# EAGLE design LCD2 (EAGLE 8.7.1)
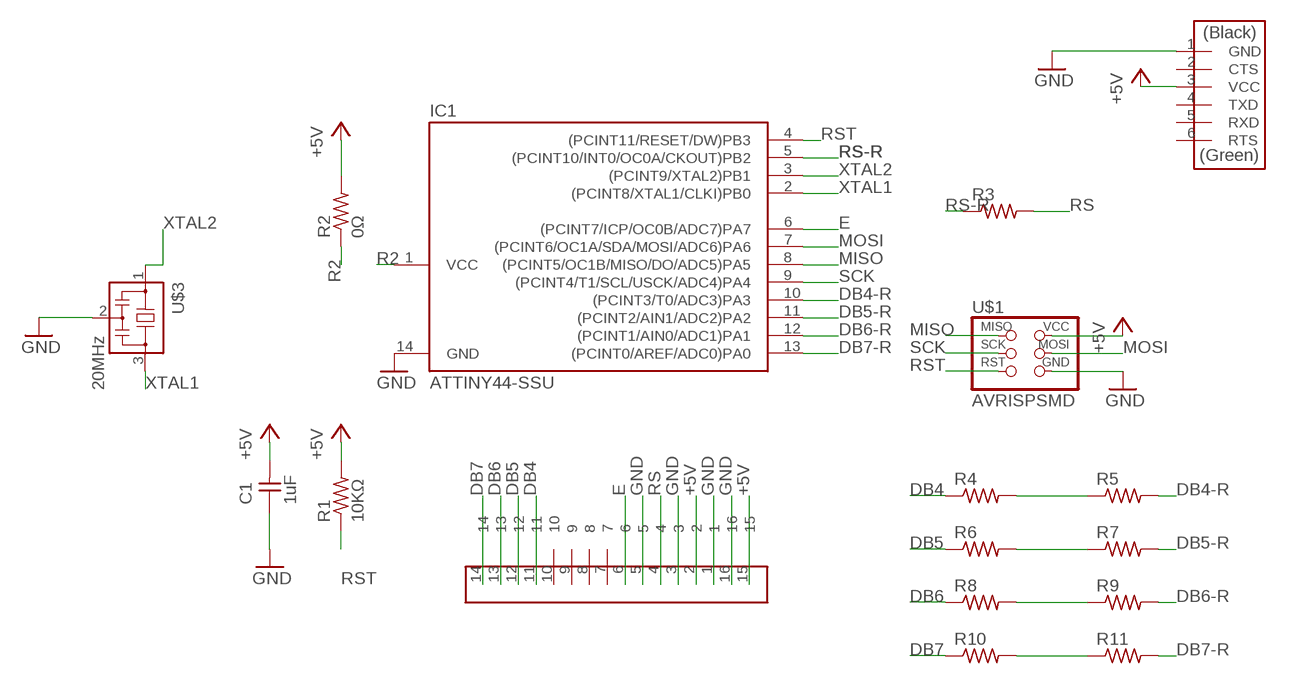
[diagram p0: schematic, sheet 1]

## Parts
C1  1uF  CAP-UNPOLARIZEDFAB  [C1206FAB]
IC1  ATTINY44-SSU  [SOIC14]
LCD1  LCD16PIN  [16PIN]
R1  10KΩ  RES-US1206FAB  [R1206FAB]
R2  0Ω  RES-US1206FAB  [R1206FAB]
R3  RES-US1206FAB  [R1206FAB]
R4  RES-US1206FAB  [R1206FAB]
R5  RES-US1206FAB  [R1206FAB]
R6  RES-US1206FAB  [R1206FAB]
R7  RES-US1206FAB  [R1206FAB]
R8  RES-US1206FAB  [R1206FAB]
R9  RES-US1206FAB  [R1206FAB]
R10  RES-US1206FAB  [R1206FAB]
R11  RES-US1206FAB  [R1206FAB]
U$1  AVRISPSMD  [2X03SMD]
U$2  FTDI-SMD-HEADER  [1X06SMD]
U$3  20MHz  RESONATOR  [EFOBM]

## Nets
+5V: C1.2 LCD1.2 LCD1.15 R1.2 R2.2 U$1.2(VCC) U$2.3(VCC)
DB4: LCD1.11 R4.1
DB4-R: IC1.10((PCINT3/T0/ADC3)PA3) R5.2
DB5: LCD1.12 R6.1
DB5-R: IC1.11((PCINT2/AIN1/ADC2)PA2) R7.2
DB6: LCD1.13 R8.1
DB6-R: IC1.12((PCINT1/AIN0/ADC1)PA1) R9.2
DB7: LCD1.14 R10.1
DB7-R: IC1.13((PCINT0/AREF/ADC0)PA0) R11.2
E: IC1.6((PCINT7/ICP/OC0B/ADC7)PA7) LCD1.6
GND: C1.1 IC1.14(GND) LCD1.1 LCD1.3 LCD1.5 LCD1.16 U$1.6(GND) U$2.1(GND) U$3.2
MISO: IC1.8((PCINT5/OC1B/MISO/DO/ADC5)PA5) U$1.1(MISO)
MOSI: IC1.7((PCINT6/OC1A/SDA/MOSI/ADC6)PA6) U$1.4(MOSI)
N$1: R4.2 R5.1
N$2: R6.2 R7.1
N$3: R8.2 R9.1
N$4: R10.2 R11.1
R2: IC1.1(VCC) R2.1
RS: LCD1.4 R3.2
RS-R: IC1.5((PCINT10/INT0/OC0A/CKOUT)PB2) R3.1
RST: IC1.4((PCINT11/RESET/DW)PB3) R1.1 U$1.5(RST)
SCK: IC1.9((PCINT4/T1/SCL/USCK/ADC4)PA4) U$1.3(SCK)
XTAL1: IC1.2((PCINT8/XTAL1/CLKI)PB0) U$3.3
XTAL2: IC1.3((PCINT9/XTAL2)PB1) U$3.1
Unconnected: LCD1.7 LCD1.8 LCD1.9 LCD1.10 U$2.2(CTS) U$2.4(TXD) U$2.5(RXD) U$2.6(RTS)

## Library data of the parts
C1 = fab:CAP-UNPOLARIZED
IC1 = fab:ATTINY44
LCD1 = doyo:LCD16PIN
R1 = fab:RES-US: Resistor (US Symbol)
R2-R11 = HelloKamakura:RES-US: Resistor (US Symbol)
U$1 = fab:AVRISP
U$2 = fab:FTDI-SMD-HEADER
U$3 = HelloKamakura:RESONATOR

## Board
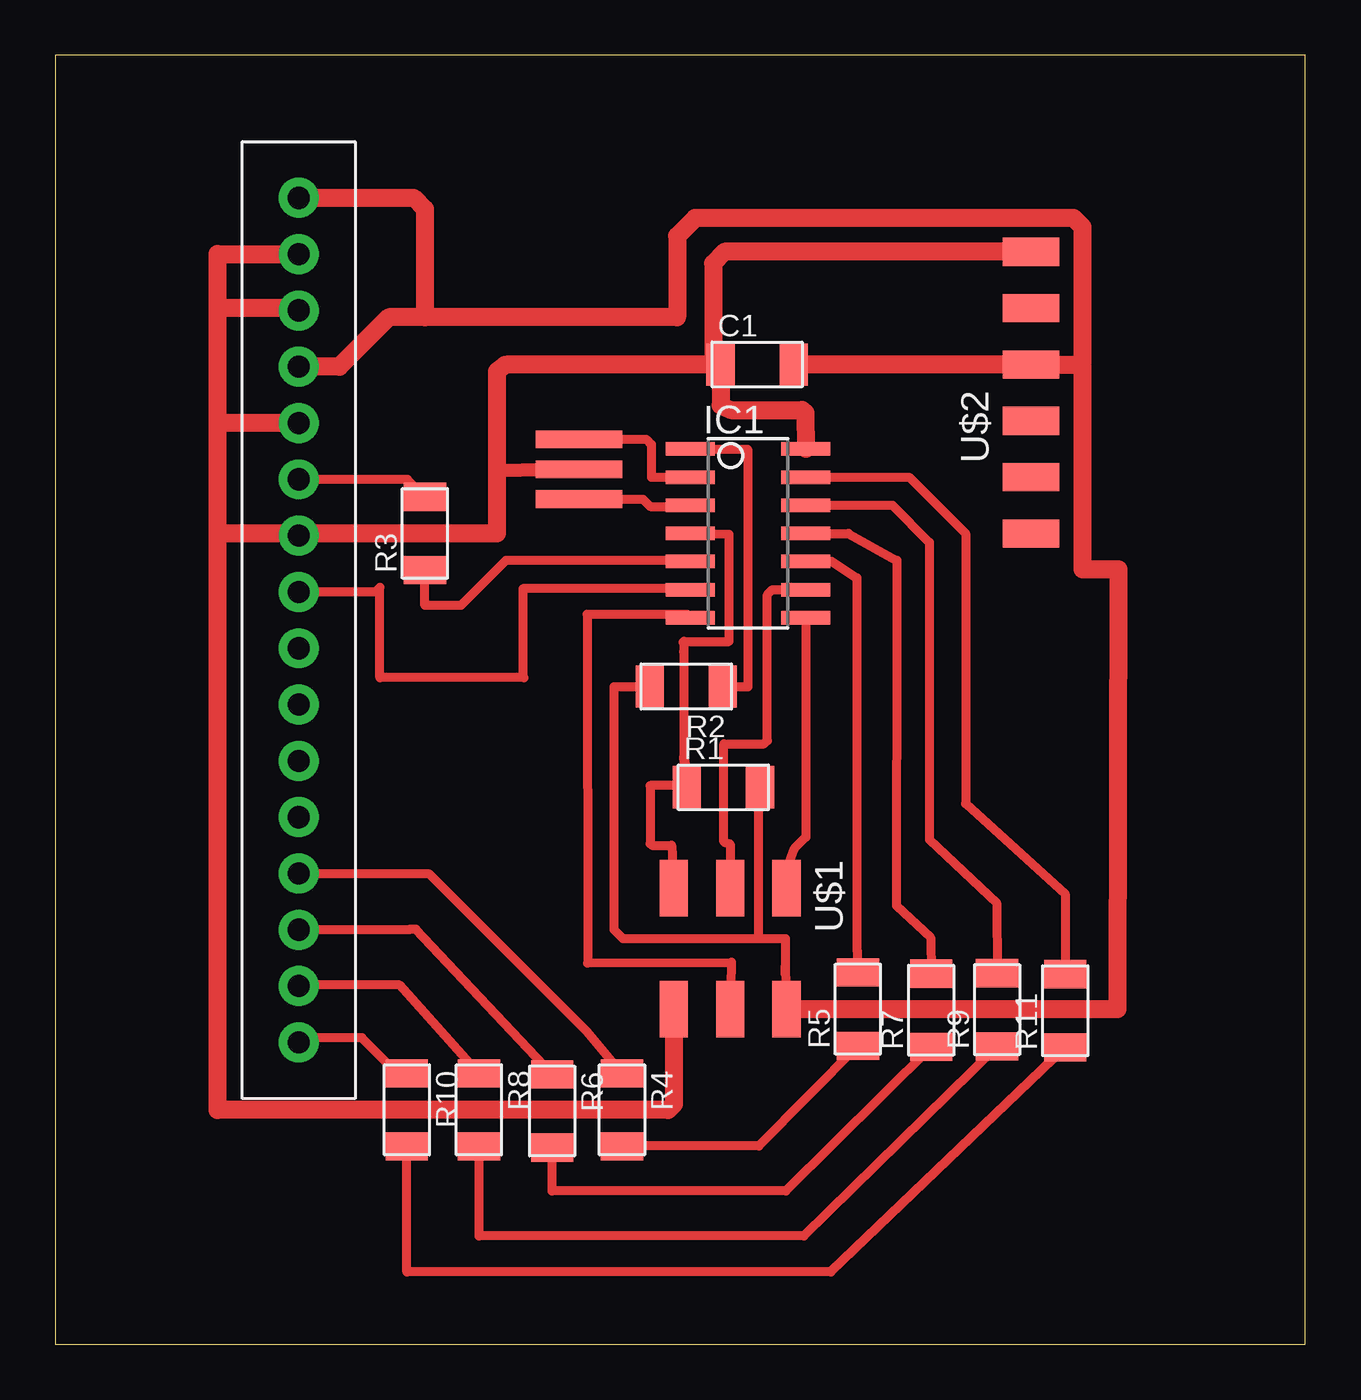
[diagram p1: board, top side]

Size 56.37 x 58.14 mm. Coordinates in mm from the lower left corner, seen from the top.
Outline: 0,0 56.37,0 56.37,58.14 0,58.14 0,0
Copper layers (1*16): Top 0.035mm / dielectric 1.5mm / Bottom 0.035mm
Design rules "default": minimum track width 6mil, minimum drill 0.35mm, track to track 6mil, track to pad 6mil, pad to pad 6mil, via to via 6mil, smd to smd 6mil, copper to edge 40mil, drill to drill 6mil, minimum pad ring 10mil, minimum via ring 8mil, stop-mask expansion 4mil, vias tented up to drill 0mil, thermal gap 10mil

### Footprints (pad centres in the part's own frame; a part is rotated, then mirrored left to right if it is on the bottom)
C1206FAB = smd 1.27 x 1.905: 1 -1.651,0; 2 1.651,0
SOIC14 = smd 0.61 x 2.21: 1 -3.81,-2.603; 2 -2.54,-2.603; 3 -1.27,-2.603; 4 0,-2.603; 5 1.27,-2.603; 6 2.54,-2.603; 7 3.81,-2.603; 8 3.81,2.603; 9 2.54,2.603; 10 1.27,2.603; 11 0,2.603; 12 -1.27,2.603; 13 -2.54,2.603; 14 -3.81,2.603
16PIN = drill 1 pad 1.8: 1 17.78,0; 2 15.24,0; 3 12.7,0; 4 10.16,0; 5 7.62,0; 6 5.08,0; 7 2.54,0; 8 0,0; 9 -2.54,0; 10 -5.08,0; 11 -7.62,0; 12 -10.16,0; 13 -12.7,0; 14 -15.24,0; 15 22.86,0; 16 20.32,0
R1206FAB = smd 1.27 x 1.905: 1 -1.651,0; 2 1.651,0
2X03SMD = smd 2.54 x 1.27: 1 -2.54,2.54; 2 2.92,2.54; 3 -2.54,0; 4 2.92,0; 5 -2.54,-2.54; 6 2.92,-2.54
1X06SMD = smd 2.54 x 1.27: 1 0,6.35; 2 0,3.81; 3 0,1.27; 4 0,-1.27; 5 0,-3.81; 6 0,-6.35
EFOBM = smd 0.8 x 3.9: 1 -1.35,0; 2 0,0; 3 1.35,0

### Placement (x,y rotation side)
C1  31.65,44.2 0 top
IC1  31.24,36.58 270 top
LCD1  10.97,28.85 90 top
R1  30.12,25.12 0 top
R2  28.45,29.67 180 top
R3  16.66,36.58 90 top
R4  25.55,10.57 270 top
R5  36.2,15.11 90 top
R6  22.4,10.52 270 top
R7  39.5,15.06 90 top
R8  19.1,10.57 270 top
R9  42.47,15.09 90 top
R10  15.85,10.57 270 top
R11  45.54,15.04 90 top
U$1  30.43,18.03 270 top
U$2  43.99,42.93 0 top
U$3  23.62,39.47 90 top

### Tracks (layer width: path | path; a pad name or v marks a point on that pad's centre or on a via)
+5V
  Top 0.406: 31.7,18.29 31.7,24.38 31.81,25.18 31.81,25.2 31.6,25.41 | 32.92,17.09 32.92,18.29 31.7,18.29 | 32.92,16.66 32.92,17.09 | 32.92,17.09 U$1.2 | R1.2 31.6,25.41 | 31.6,25.41 31.62,24.99 | 31.7,18.29 25.6,18.29 25.2,18.69 25.2,29.67 R2.2
  Top 0.813: C1.2 U$2.3 46.23,44.2 | 46.23,44.2 46.33,44.3 46.33,50.39 45.92,50.8 28.85,50.8 28.04,49.99 28.04,46.33 16.66,46.33 | 16.66,46.33 15.04,46.33 12.8,44.09 LCD1.2 | U$1.2 37.47,15.11 47.9,15.11 47.95,34.95 46.33,34.95 46.33,44.09 46.23,44.2 | LCD1.15 16.15,51.71 16.66,51.21 16.66,46.33
DB4
  Top 0.406: R4.1 23.98,14.1 16.87,21.21 11,21.21 LCD1.11
DB4-R
  Top 0.406: IC1.10 35,35.31 36.14,34.57 36.14,17.75 36.17,17.73 R5.2
DB5
  Top 0.406: R6.1 16.26,18.72 16,18.72 15.98,18.69 LCD1.12
DB5-R
  Top 0.406: IC1.11 35.76,36.58 37.95,35.36 37.95,32.92 37.92,19.79 39.47,18.34 R7.2
DB6
  Top 0.406: R8.1 15.52,16.2 11.02,16.2 LCD1.13
DB6-R
  Top 0.406: IC1.12 37.74,37.85 39.42,36.17 39.42,22.76 42.44,19.91 R9.2
DB7
  Top 0.406: R10.1 15.42,12.22 13.82,13.82 11.18,13.82 LCD1.14
DB7-R
  Top 0.406: IC1.13 38.51,39.12 41.05,36.58 41.05,24.38 45.54,20.32 R11.2
E
  Top 0.406: IC1.6 28.59,34.09 21.08,34.09 21.08,30.12 21.13,30.07 14.63,30.07 14.63,34.14 14.43,33.93 LCD1.6
GND
  Top 0.61: 19.91,39.42 23.19,39.47 | 11.07,36.58 LCD1.5
  Top 0.813: U$2.1 30.18,49.28 29.67,48.77 29.67,44.27 C1.1 | C1.1 20.42,44.2 20.27,44.17 19.91,43.89 19.91,39.42 19.91,36.58 11.07,36.58 | 23.19,39.47 U$3.2 | 27.71,15.52 U$1.6 27.89,10.82 27.64,10.57 7.32,10.57 7.32,36.58 | C1.1 30,42.34 30.45,42.14 33.68,42.14 33.82,42.02 IC1.14 | 7.42,36.47 7.32,36.58 | 7.32,41.45 7.32,46.74 | 7.32,46.74 7.32,49.17 LCD1.16 | LCD1.1 10.87,46.74 7.32,46.74 | LCD1.3 7.42,41.55 7.32,41.45 | LCD1.5 10.87,36.58 7.32,36.58 | 7.32,36.58 7.32,41.45
MISO
  Top 0.406: IC1.8 33.85,22.87 33.33,22.35 32.66,20.57 U$1.1
MOSI
  Top 0.406: IC1.7 28.49,32.92 23.98,32.92 24,17.2 30.48,17.22 30.48,17.2 U$1.4
N$1
  Top 0.406: R5.1 31.73,8.94 25.63,8.94 R4.2
N$2
  Top 0.406: R7.1 32.94,6.91 22.4,6.91 R6.2
N$3
  Top 0.406: R9.1 33.76,4.88 19.1,4.88 R8.2
N$4
  Top 0.406: R11.1 34.98,3.25 15.85,3.25 R10.2
R2
  Top 0.406: R2.1 31.24,29.67 31.24,40.28 31.22,40.36 28.66,40.36 IC1.1
RS
  Top 0.406: R3.2 15.88,39.01 LCD1.4
RS-R
  Top 0.406: IC1.5 28.59,35.36 20.32,35.36 18.29,33.33 16.66,33.33 R3.1
RST
  Top 0.406: 28.33,26.48 R1.1 28.4,25.2 26.82,25.2 26.82,22.58 26.9,22.5 27.79,22.5 U$1.5 | 28.33,26.48 28.45,25.93 | 28.3,31.67 28.34,31.71 | 28.34,31.71 30.38,31.7 30.38,36.52 28.66,36.55 IC1.4 | 28.34,31.71 28.33,31.24 28.33,26.48
SCK
  Top 0.406: U$1.3 30.43,22.55 30.15,22.66 30.15,27.08 31.95,27.08 32.11,27.23 32.11,33.81 32.33,34.04 IC1.9
XTAL1
  Top 0.406: U$3.3 26.64,40.82 26.87,40.59 26.87,39.12 IC1.2
XTAL2
  Top 0.406: U$3.1 26.5,38.12 26.82,37.8 28.59,37.8 IC1.3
